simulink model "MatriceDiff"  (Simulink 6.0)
settings: Solver=ode45  StartTime=0  StopTime=17*t0  RelTol=1e-3
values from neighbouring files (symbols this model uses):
  b = S/Sm    (= 0.1)    [Constantes.m]    (also in ConstantesBck.m)
  beta = 0.95    [Constantes.m]    (also in ConstantesBck.m; ResCourV1.m = 1; ResCrV1.m = 1; ResEnerV1.m = 1)
  C = 1    [Constantes.m]    (also in ConstantesBck.m)
  gk = 36    [Constantes.m]    (also in ConstantesBck.m; sim_hh.m)
  gl = 0.3    [Constantes.m]    (also in ConstantesBck.m; sim_hh.m)
  gna = 120    [Constantes.m]    (also in ConstantesBck.m; sim_hh.m)
  h0 = 0.5961    [Constantes.m]    (also in ConstantesBck.m)
  m0 = 0.0529    [Constantes.m]    (also in ConstantesBck.m)
  mK = 0    [Constantes.m]    (also in ConstantesBck.m)
  mL = 0    [Constantes.m]    (also in ConstantesBck.m)
  mNa = 0    [Constantes.m]    (also in ConstantesBck.m)
  N = [6,8,5,5,7,1,2,6,9,1,1,9,4,8,8,7]    [Constantes.m]    (also in ConstantesBck.m; ImpedanceZtissus.m = 100; Ztissus.m = 100; charge.m = N(:,2))
  n0 = 0.3177    [Constantes.m]    (also in ConstantesBck.m)
  rapportIE = 10    [Constantes.m]
  Sm = 3.14e-2    (= 0.0314)    [Constantes.m]    (also in ConstantesBck.m = 0.000314)
  t0 = 2E-3    (= 0.002)    [Constantes.m]    (also in ConstantesBck.m = 0.001)
  Vk = -82    [Constantes.m]    (also in ConstantesBck.m)
  Vl = -59    [Constantes.m]    (also in ConstantesBck.m)
  Vna = 45    [Constantes.m]    (also in ConstantesBck.m)
  Vr = -70    [Constantes.m]    (also in ConstantesBck.m)
undefined symbols (not defined in the file or in its folder): ln
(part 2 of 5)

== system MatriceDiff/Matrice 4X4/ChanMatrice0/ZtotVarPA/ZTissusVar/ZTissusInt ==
  InStim : Inport  Orientation=down  Port=1  LatchInput=off
  VRefIn : Inport  Port=2  LatchInput=off
  Constant : Constant  Value=0
  Gain2 : Gain  Gain=-1
  Gain3 : Gain  Gain=-1
  Gain4 : Gain  Gain=-1
  Modele HH : Subsystem
  Modele HH1 : Subsystem
  Rint : Fcn  Expr=u*(1.6342*((abs(u)*1E6)^0.1267))*1E3/rapportIE
  Sum1 : Sum  Inputs=|+++
  Vout : Outport
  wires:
  Modele HH1/1(HHout) -> Gain3/1
  Modele HH/1(HHout) -> Gain4/1
  Rint/1 -> Sum1/2
  Gain2/1 -> Modele HH/1(HHin)
  InStim/1 -> Gain2/1, Rint/1, Modele HH1/1(HHin)
  Constant/1 -> Modele HH1/2(VRefIn)
  Sum1/1 -> Vout/1
  VRefIn/1 -> Modele HH/2(VRefIn)
  Gain3/1 -> Sum1/1
  Gain4/1 -> Sum1/3

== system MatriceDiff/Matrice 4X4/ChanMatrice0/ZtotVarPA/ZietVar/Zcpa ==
  InZcpa : Inport  Port=1  LatchInput=off
  Cdl : Fcn  Expr=u*1E9/(918.15-80.854*ln(abs(u)*1E6))
  Fcn : Fcn  Expr=u(1)^beta
  Transfer Fcn : TransferFcn  Denominator=[1 0]
  OutZcpa : Outport
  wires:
  Transfer Fcn/1 -> Fcn/1
  InZcpa/1 -> Cdl/1
  Fcn/1 -> OutZcpa/1
  Cdl/1 -> Transfer Fcn/1

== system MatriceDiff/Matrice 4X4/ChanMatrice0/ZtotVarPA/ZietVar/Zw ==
  InZw : Inport  Port=1  LatchInput=off
  Math Function : Math  Operator=sqrt
  Product : Product
  Transfer Fcn : TransferFcn  Numerator=[2]  Denominator=[1 0]
  sigma : Fcn  Expr=(67202-0.0688*((1E6*abs(u))^2)-11.273*(1E6*abs(u)))
  OutZw : Outport
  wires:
  Transfer Fcn/1 -> Math Function/1
  InZw/1 -> Transfer Fcn/1, sigma/1
  Math Function/1 -> Product/1
  sigma/1 -> Product/2
  Product/1 -> OutZw/1

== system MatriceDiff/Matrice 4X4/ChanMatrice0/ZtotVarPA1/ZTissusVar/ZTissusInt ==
  InStim : Inport  Orientation=down  Port=1  LatchInput=off
  VRefIn : Inport  Port=2  LatchInput=off
  Constant : Constant  Value=0
  Gain2 : Gain  Gain=-1
  Gain3 : Gain  Gain=-1
  Gain4 : Gain  Gain=-1
  Modele HH : Subsystem
  Modele HH1 : Subsystem
  Rint : Fcn  Expr=u*(1.6342*((abs(u)*1E6)^0.1267))*1E3/rapportIE
  Sum1 : Sum  Inputs=|+++
  Vout : Outport
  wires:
  Modele HH1/1(HHout) -> Gain3/1
  Modele HH/1(HHout) -> Gain4/1
  Rint/1 -> Sum1/2
  Gain2/1 -> Modele HH/1(HHin)
  InStim/1 -> Gain2/1, Rint/1, Modele HH1/1(HHin)
  Constant/1 -> Modele HH1/2(VRefIn)
  Sum1/1 -> Vout/1
  VRefIn/1 -> Modele HH/2(VRefIn)
  Gain3/1 -> Sum1/1
  Gain4/1 -> Sum1/3

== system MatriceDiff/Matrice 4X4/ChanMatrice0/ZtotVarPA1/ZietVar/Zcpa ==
  InZcpa : Inport  Port=1  LatchInput=off
  Cdl : Fcn  Expr=u*1E9/(918.15-80.854*ln(abs(u)*1E6))
  Fcn : Fcn  Expr=u(1)^beta
  Transfer Fcn : TransferFcn  Denominator=[1 0]
  OutZcpa : Outport
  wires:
  Transfer Fcn/1 -> Fcn/1
  InZcpa/1 -> Cdl/1
  Fcn/1 -> OutZcpa/1
  Cdl/1 -> Transfer Fcn/1

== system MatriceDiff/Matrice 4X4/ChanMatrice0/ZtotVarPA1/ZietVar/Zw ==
  InZw : Inport  Port=1  LatchInput=off
  Math Function : Math  Operator=sqrt
  Product : Product
  Transfer Fcn : TransferFcn  Numerator=[2]  Denominator=[1 0]
  sigma : Fcn  Expr=(67202-0.0688*((1E6*abs(u))^2)-11.273*(1E6*abs(u)))
  OutZw : Outport
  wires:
  Transfer Fcn/1 -> Math Function/1
  InZw/1 -> Transfer Fcn/1, sigma/1
  Math Function/1 -> Product/1
  sigma/1 -> Product/2
  Product/1 -> OutZw/1

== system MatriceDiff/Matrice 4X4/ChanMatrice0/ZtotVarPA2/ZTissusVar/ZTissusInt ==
  InStim : Inport  Orientation=down  Port=1  LatchInput=off
  VRefIn : Inport  Port=2  LatchInput=off
  Constant : Constant  Value=0
  Gain2 : Gain  Gain=-1
  Gain3 : Gain  Gain=-1
  Gain4 : Gain  Gain=-1
  Modele HH : Subsystem
  Modele HH1 : Subsystem
  Rint : Fcn  Expr=u*(1.6342*((abs(u)*1E6)^0.1267))*1E3/rapportIE
  Sum1 : Sum  Inputs=|+++
  Vout : Outport
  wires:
  Modele HH1/1(HHout) -> Gain3/1
  Modele HH/1(HHout) -> Gain4/1
  Rint/1 -> Sum1/2
  Gain2/1 -> Modele HH/1(HHin)
  InStim/1 -> Gain2/1, Rint/1, Modele HH1/1(HHin)
  Constant/1 -> Modele HH1/2(VRefIn)
  Sum1/1 -> Vout/1
  VRefIn/1 -> Modele HH/2(VRefIn)
  Gain3/1 -> Sum1/1
  Gain4/1 -> Sum1/3

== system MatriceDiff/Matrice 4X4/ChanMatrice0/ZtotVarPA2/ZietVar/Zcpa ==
  InZcpa : Inport  Port=1  LatchInput=off
  Cdl : Fcn  Expr=u*1E9/(918.15-80.854*ln(abs(u)*1E6))
  Fcn : Fcn  Expr=u(1)^beta
  Transfer Fcn : TransferFcn  Denominator=[1 0]
  OutZcpa : Outport
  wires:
  Transfer Fcn/1 -> Fcn/1
  InZcpa/1 -> Cdl/1
  Fcn/1 -> OutZcpa/1
  Cdl/1 -> Transfer Fcn/1

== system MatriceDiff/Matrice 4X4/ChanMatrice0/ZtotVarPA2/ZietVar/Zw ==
  InZw : Inport  Port=1  LatchInput=off
  Math Function : Math  Operator=sqrt
  Product : Product
  Transfer Fcn : TransferFcn  Numerator=[2]  Denominator=[1 0]
  sigma : Fcn  Expr=(67202-0.0688*((1E6*abs(u))^2)-11.273*(1E6*abs(u)))
  OutZw : Outport
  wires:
  Transfer Fcn/1 -> Math Function/1
  InZw/1 -> Transfer Fcn/1, sigma/1
  Math Function/1 -> Product/1
  sigma/1 -> Product/2
  Product/1 -> OutZw/1

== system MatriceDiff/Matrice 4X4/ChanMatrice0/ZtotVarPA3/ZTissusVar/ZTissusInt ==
  InStim : Inport  Orientation=down  Port=1  LatchInput=off
  VRefIn : Inport  Port=2  LatchInput=off
  Constant : Constant  Value=0
  Gain2 : Gain  Gain=-1
  Gain3 : Gain  Gain=-1
  Gain4 : Gain  Gain=-1
  Modele HH : Subsystem
  Modele HH1 : Subsystem
  Rint : Fcn  Expr=u*(1.6342*((abs(u)*1E6)^0.1267))*1E3/rapportIE
  Sum1 : Sum  Inputs=|+++
  Vout : Outport
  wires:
  Modele HH1/1(HHout) -> Gain3/1
  Modele HH/1(HHout) -> Gain4/1
  Rint/1 -> Sum1/2
  Gain2/1 -> Modele HH/1(HHin)
  InStim/1 -> Gain2/1, Rint/1, Modele HH1/1(HHin)
  Constant/1 -> Modele HH1/2(VRefIn)
  Sum1/1 -> Vout/1
  VRefIn/1 -> Modele HH/2(VRefIn)
  Gain3/1 -> Sum1/1
  Gain4/1 -> Sum1/3

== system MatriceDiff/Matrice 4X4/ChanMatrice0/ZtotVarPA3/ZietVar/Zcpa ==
  InZcpa : Inport  Port=1  LatchInput=off
  Cdl : Fcn  Expr=u*1E9/(918.15-80.854*ln(abs(u)*1E6))
  Fcn : Fcn  Expr=u(1)^beta
  Transfer Fcn : TransferFcn  Denominator=[1 0]
  OutZcpa : Outport
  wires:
  Transfer Fcn/1 -> Fcn/1
  InZcpa/1 -> Cdl/1
  Fcn/1 -> OutZcpa/1
  Cdl/1 -> Transfer Fcn/1

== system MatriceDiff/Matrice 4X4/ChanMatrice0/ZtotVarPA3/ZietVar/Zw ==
  InZw : Inport  Port=1  LatchInput=off
  Math Function : Math  Operator=sqrt
  Product : Product
  Transfer Fcn : TransferFcn  Numerator=[2]  Denominator=[1 0]
  sigma : Fcn  Expr=(67202-0.0688*((1E6*abs(u))^2)-11.273*(1E6*abs(u)))
  OutZw : Outport
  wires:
  Transfer Fcn/1 -> Math Function/1
  InZw/1 -> Transfer Fcn/1, sigma/1
  Math Function/1 -> Product/1
  sigma/1 -> Product/2
  Product/1 -> OutZw/1

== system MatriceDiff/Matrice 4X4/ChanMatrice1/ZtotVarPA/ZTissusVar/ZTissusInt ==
  InStim : Inport  Orientation=down  Port=1  LatchInput=off
  VRefIn : Inport  Port=2  LatchInput=off
  Constant : Constant  Value=0
  Gain2 : Gain  Gain=-1
  Gain3 : Gain  Gain=-1
  Gain4 : Gain  Gain=-1
  Modele HH : Subsystem
  Modele HH1 : Subsystem
  Rint : Fcn  Expr=u*(1.6342*((abs(u)*1E6)^0.1267))*1E3/rapportIE
  Sum1 : Sum  Inputs=|+++
  Vout : Outport
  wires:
  Modele HH1/1(HHout) -> Gain3/1
  Modele HH/1(HHout) -> Gain4/1
  Rint/1 -> Sum1/2
  Gain2/1 -> Modele HH/1(HHin)
  InStim/1 -> Gain2/1, Rint/1, Modele HH1/1(HHin)
  Constant/1 -> Modele HH1/2(VRefIn)
  Sum1/1 -> Vout/1
  VRefIn/1 -> Modele HH/2(VRefIn)
  Gain3/1 -> Sum1/1
  Gain4/1 -> Sum1/3

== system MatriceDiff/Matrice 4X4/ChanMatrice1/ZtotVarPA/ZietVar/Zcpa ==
  InZcpa : Inport  Port=1  LatchInput=off
  Cdl : Fcn  Expr=u*1E9/(918.15-80.854*ln(abs(u)*1E6))
  Fcn : Fcn  Expr=u(1)^beta
  Transfer Fcn : TransferFcn  Denominator=[1 0]
  OutZcpa : Outport
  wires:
  Transfer Fcn/1 -> Fcn/1
  InZcpa/1 -> Cdl/1
  Fcn/1 -> OutZcpa/1
  Cdl/1 -> Transfer Fcn/1

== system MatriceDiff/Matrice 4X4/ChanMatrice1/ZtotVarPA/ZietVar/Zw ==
  InZw : Inport  Port=1  LatchInput=off
  Math Function : Math  Operator=sqrt
  Product : Product
  Transfer Fcn : TransferFcn  Numerator=[2]  Denominator=[1 0]
  sigma : Fcn  Expr=(67202-0.0688*((1E6*abs(u))^2)-11.273*(1E6*abs(u)))
  OutZw : Outport
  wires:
  Transfer Fcn/1 -> Math Function/1
  InZw/1 -> Transfer Fcn/1, sigma/1
  Math Function/1 -> Product/1
  sigma/1 -> Product/2
  Product/1 -> OutZw/1

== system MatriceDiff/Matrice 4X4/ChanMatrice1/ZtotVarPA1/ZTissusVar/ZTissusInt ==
  InStim : Inport  Orientation=down  Port=1  LatchInput=off
  VRefIn : Inport  Port=2  LatchInput=off
  Constant : Constant  Value=0
  Gain2 : Gain  Gain=-1
  Gain3 : Gain  Gain=-1
  Gain4 : Gain  Gain=-1
  Modele HH : Subsystem
  Modele HH1 : Subsystem
  Rint : Fcn  Expr=u*(1.6342*((abs(u)*1E6)^0.1267))*1E3/rapportIE
  Sum1 : Sum  Inputs=|+++
  Vout : Outport
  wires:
  Modele HH1/1(HHout) -> Gain3/1
  Modele HH/1(HHout) -> Gain4/1
  Rint/1 -> Sum1/2
  Gain2/1 -> Modele HH/1(HHin)
  InStim/1 -> Gain2/1, Rint/1, Modele HH1/1(HHin)
  Constant/1 -> Modele HH1/2(VRefIn)
  Sum1/1 -> Vout/1
  VRefIn/1 -> Modele HH/2(VRefIn)
  Gain3/1 -> Sum1/1
  Gain4/1 -> Sum1/3

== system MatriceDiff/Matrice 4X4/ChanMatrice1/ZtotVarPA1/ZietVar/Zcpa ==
  InZcpa : Inport  Port=1  LatchInput=off
  Cdl : Fcn  Expr=u*1E9/(918.15-80.854*ln(abs(u)*1E6))
  Fcn : Fcn  Expr=u(1)^beta
  Transfer Fcn : TransferFcn  Denominator=[1 0]
  OutZcpa : Outport
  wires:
  Transfer Fcn/1 -> Fcn/1
  InZcpa/1 -> Cdl/1
  Fcn/1 -> OutZcpa/1
  Cdl/1 -> Transfer Fcn/1

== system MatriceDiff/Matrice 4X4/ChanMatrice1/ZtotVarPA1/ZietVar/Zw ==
  InZw : Inport  Port=1  LatchInput=off
  Math Function : Math  Operator=sqrt
  Product : Product
  Transfer Fcn : TransferFcn  Numerator=[2]  Denominator=[1 0]
  sigma : Fcn  Expr=(67202-0.0688*((1E6*abs(u))^2)-11.273*(1E6*abs(u)))
  OutZw : Outport
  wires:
  Transfer Fcn/1 -> Math Function/1
  InZw/1 -> Transfer Fcn/1, sigma/1
  Math Function/1 -> Product/1
  sigma/1 -> Product/2
  Product/1 -> OutZw/1

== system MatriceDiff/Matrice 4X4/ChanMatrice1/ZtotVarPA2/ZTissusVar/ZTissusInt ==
  InStim : Inport  Orientation=down  Port=1  LatchInput=off
  VRefIn : Inport  Port=2  LatchInput=off
  Constant : Constant  Value=0
  Gain2 : Gain  Gain=-1
  Gain3 : Gain  Gain=-1
  Gain4 : Gain  Gain=-1
  Modele HH : Subsystem
  Modele HH1 : Subsystem
  Rint : Fcn  Expr=u*(1.6342*((abs(u)*1E6)^0.1267))*1E3/rapportIE
  Sum1 : Sum  Inputs=|+++
  Vout : Outport
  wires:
  Modele HH1/1(HHout) -> Gain3/1
  Modele HH/1(HHout) -> Gain4/1
  Rint/1 -> Sum1/2
  Gain2/1 -> Modele HH/1(HHin)
  InStim/1 -> Gain2/1, Rint/1, Modele HH1/1(HHin)
  Constant/1 -> Modele HH1/2(VRefIn)
  Sum1/1 -> Vout/1
  VRefIn/1 -> Modele HH/2(VRefIn)
  Gain3/1 -> Sum1/1
  Gain4/1 -> Sum1/3

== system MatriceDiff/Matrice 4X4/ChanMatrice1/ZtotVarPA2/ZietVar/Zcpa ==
  InZcpa : Inport  Port=1  LatchInput=off
  Cdl : Fcn  Expr=u*1E9/(918.15-80.854*ln(abs(u)*1E6))
  Fcn : Fcn  Expr=u(1)^beta
  Transfer Fcn : TransferFcn  Denominator=[1 0]
  OutZcpa : Outport
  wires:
  Transfer Fcn/1 -> Fcn/1
  InZcpa/1 -> Cdl/1
  Fcn/1 -> OutZcpa/1
  Cdl/1 -> Transfer Fcn/1

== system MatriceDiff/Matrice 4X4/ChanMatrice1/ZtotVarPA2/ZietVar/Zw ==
  InZw : Inport  Port=1  LatchInput=off
  Math Function : Math  Operator=sqrt
  Product : Product
  Transfer Fcn : TransferFcn  Numerator=[2]  Denominator=[1 0]
  sigma : Fcn  Expr=(67202-0.0688*((1E6*abs(u))^2)-11.273*(1E6*abs(u)))
  OutZw : Outport
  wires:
  Transfer Fcn/1 -> Math Function/1
  InZw/1 -> Transfer Fcn/1, sigma/1
  Math Function/1 -> Product/1
  sigma/1 -> Product/2
  Product/1 -> OutZw/1

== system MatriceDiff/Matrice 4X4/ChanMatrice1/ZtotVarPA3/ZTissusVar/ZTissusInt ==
  InStim : Inport  Orientation=down  Port=1  LatchInput=off
  VRefIn : Inport  Port=2  LatchInput=off
  Constant : Constant  Value=0
  Gain2 : Gain  Gain=-1
  Gain3 : Gain  Gain=-1
  Gain4 : Gain  Gain=-1
  Modele HH : Subsystem
  Modele HH1 : Subsystem
  Rint : Fcn  Expr=u*(1.6342*((abs(u)*1E6)^0.1267))*1E3/rapportIE
  Sum1 : Sum  Inputs=|+++
  Vout : Outport
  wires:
  Modele HH1/1(HHout) -> Gain3/1
  Modele HH/1(HHout) -> Gain4/1
  Rint/1 -> Sum1/2
  Gain2/1 -> Modele HH/1(HHin)
  InStim/1 -> Gain2/1, Rint/1, Modele HH1/1(HHin)
  Constant/1 -> Modele HH1/2(VRefIn)
  Sum1/1 -> Vout/1
  VRefIn/1 -> Modele HH/2(VRefIn)
  Gain3/1 -> Sum1/1
  Gain4/1 -> Sum1/3

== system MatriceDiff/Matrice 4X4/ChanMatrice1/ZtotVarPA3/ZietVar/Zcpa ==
  InZcpa : Inport  Port=1  LatchInput=off
  Cdl : Fcn  Expr=u*1E9/(918.15-80.854*ln(abs(u)*1E6))
  Fcn : Fcn  Expr=u(1)^beta
  Transfer Fcn : TransferFcn  Denominator=[1 0]
  OutZcpa : Outport
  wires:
  Transfer Fcn/1 -> Fcn/1
  InZcpa/1 -> Cdl/1
  Fcn/1 -> OutZcpa/1
  Cdl/1 -> Transfer Fcn/1

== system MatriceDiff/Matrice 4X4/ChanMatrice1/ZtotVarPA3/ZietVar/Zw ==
  InZw : Inport  Port=1  LatchInput=off
  Math Function : Math  Operator=sqrt
  Product : Product
  Transfer Fcn : TransferFcn  Numerator=[2]  Denominator=[1 0]
  sigma : Fcn  Expr=(67202-0.0688*((1E6*abs(u))^2)-11.273*(1E6*abs(u)))
  OutZw : Outport
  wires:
  Transfer Fcn/1 -> Math Function/1
  InZw/1 -> Transfer Fcn/1, sigma/1
  Math Function/1 -> Product/1
  sigma/1 -> Product/2
  Product/1 -> OutZw/1

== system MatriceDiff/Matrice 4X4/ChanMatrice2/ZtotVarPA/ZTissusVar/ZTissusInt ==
  InStim : Inport  Orientation=down  Port=1  LatchInput=off
  VRefIn : Inport  Port=2  LatchInput=off
  Constant : Constant  Value=0
  Gain2 : Gain  Gain=-1
  Gain3 : Gain  Gain=-1
  Gain4 : Gain  Gain=-1
  Modele HH : Subsystem
  Modele HH1 : Subsystem
  Rint : Fcn  Expr=u*(1.6342*((abs(u)*1E6)^0.1267))*1E3/rapportIE
  Sum1 : Sum  Inputs=|+++
  Vout : Outport
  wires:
  Modele HH1/1(HHout) -> Gain3/1
  Modele HH/1(HHout) -> Gain4/1
  Rint/1 -> Sum1/2
  Gain2/1 -> Modele HH/1(HHin)
  InStim/1 -> Gain2/1, Rint/1, Modele HH1/1(HHin)
  Constant/1 -> Modele HH1/2(VRefIn)
  Sum1/1 -> Vout/1
  VRefIn/1 -> Modele HH/2(VRefIn)
  Gain3/1 -> Sum1/1
  Gain4/1 -> Sum1/3

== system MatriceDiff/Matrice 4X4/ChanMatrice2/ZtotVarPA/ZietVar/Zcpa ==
  InZcpa : Inport  Port=1  LatchInput=off
  Cdl : Fcn  Expr=u*1E9/(918.15-80.854*ln(abs(u)*1E6))
  Fcn : Fcn  Expr=u(1)^beta
  Transfer Fcn : TransferFcn  Denominator=[1 0]
  OutZcpa : Outport
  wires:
  Transfer Fcn/1 -> Fcn/1
  InZcpa/1 -> Cdl/1
  Fcn/1 -> OutZcpa/1
  Cdl/1 -> Transfer Fcn/1

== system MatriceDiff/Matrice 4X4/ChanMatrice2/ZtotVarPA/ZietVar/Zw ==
  InZw : Inport  Port=1  LatchInput=off
  Math Function : Math  Operator=sqrt
  Product : Product
  Transfer Fcn : TransferFcn  Numerator=[2]  Denominator=[1 0]
  sigma : Fcn  Expr=(67202-0.0688*((1E6*abs(u))^2)-11.273*(1E6*abs(u)))
  OutZw : Outport
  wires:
  Transfer Fcn/1 -> Math Function/1
  InZw/1 -> Transfer Fcn/1, sigma/1
  Math Function/1 -> Product/1
  sigma/1 -> Product/2
  Product/1 -> OutZw/1

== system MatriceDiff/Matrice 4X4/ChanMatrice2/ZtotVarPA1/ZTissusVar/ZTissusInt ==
  InStim : Inport  Orientation=down  Port=1  LatchInput=off
  VRefIn : Inport  Port=2  LatchInput=off
  Constant : Constant  Value=0
  Gain2 : Gain  Gain=-1
  Gain3 : Gain  Gain=-1
  Gain4 : Gain  Gain=-1
  Modele HH : Subsystem
  Modele HH1 : Subsystem
  Rint : Fcn  Expr=u*(1.6342*((abs(u)*1E6)^0.1267))*1E3/rapportIE
  Sum1 : Sum  Inputs=|+++
  Vout : Outport
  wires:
  Modele HH1/1(HHout) -> Gain3/1
  Modele HH/1(HHout) -> Gain4/1
  Rint/1 -> Sum1/2
  Gain2/1 -> Modele HH/1(HHin)
  InStim/1 -> Gain2/1, Rint/1, Modele HH1/1(HHin)
  Constant/1 -> Modele HH1/2(VRefIn)
  Sum1/1 -> Vout/1
  VRefIn/1 -> Modele HH/2(VRefIn)
  Gain3/1 -> Sum1/1
  Gain4/1 -> Sum1/3

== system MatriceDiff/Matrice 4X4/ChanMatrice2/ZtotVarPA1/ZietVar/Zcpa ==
  InZcpa : Inport  Port=1  LatchInput=off
  Cdl : Fcn  Expr=u*1E9/(918.15-80.854*ln(abs(u)*1E6))
  Fcn : Fcn  Expr=u(1)^beta
  Transfer Fcn : TransferFcn  Denominator=[1 0]
  OutZcpa : Outport
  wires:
  Transfer Fcn/1 -> Fcn/1
  InZcpa/1 -> Cdl/1
  Fcn/1 -> OutZcpa/1
  Cdl/1 -> Transfer Fcn/1

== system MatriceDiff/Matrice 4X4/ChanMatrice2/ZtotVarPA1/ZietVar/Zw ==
  InZw : Inport  Port=1  LatchInput=off
  Math Function : Math  Operator=sqrt
  Product : Product
  Transfer Fcn : TransferFcn  Numerator=[2]  Denominator=[1 0]
  sigma : Fcn  Expr=(67202-0.0688*((1E6*abs(u))^2)-11.273*(1E6*abs(u)))
  OutZw : Outport
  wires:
  Transfer Fcn/1 -> Math Function/1
  InZw/1 -> Transfer Fcn/1, sigma/1
  Math Function/1 -> Product/1
  sigma/1 -> Product/2
  Product/1 -> OutZw/1

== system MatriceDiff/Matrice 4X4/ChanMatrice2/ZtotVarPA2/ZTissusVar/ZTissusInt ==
  InStim : Inport  Orientation=down  Port=1  LatchInput=off
  VRefIn : Inport  Port=2  LatchInput=off
  Constant : Constant  Value=0
  Gain2 : Gain  Gain=-1
  Gain3 : Gain  Gain=-1
  Gain4 : Gain  Gain=-1
  Modele HH : Subsystem
  Modele HH1 : Subsystem
  Rint : Fcn  Expr=u*(1.6342*((abs(u)*1E6)^0.1267))*1E3/rapportIE
  Sum1 : Sum  Inputs=|+++
  Vout : Outport
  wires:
  Modele HH1/1(HHout) -> Gain3/1
  Modele HH/1(HHout) -> Gain4/1
  Rint/1 -> Sum1/2
  Gain2/1 -> Modele HH/1(HHin)
  InStim/1 -> Gain2/1, Rint/1, Modele HH1/1(HHin)
  Constant/1 -> Modele HH1/2(VRefIn)
  Sum1/1 -> Vout/1
  VRefIn/1 -> Modele HH/2(VRefIn)
  Gain3/1 -> Sum1/1
  Gain4/1 -> Sum1/3

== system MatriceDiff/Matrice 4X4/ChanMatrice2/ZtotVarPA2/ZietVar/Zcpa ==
  InZcpa : Inport  Port=1  LatchInput=off
  Cdl : Fcn  Expr=u*1E9/(918.15-80.854*ln(abs(u)*1E6))
  Fcn : Fcn  Expr=u(1)^beta
  Transfer Fcn : TransferFcn  Denominator=[1 0]
  OutZcpa : Outport
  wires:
  Transfer Fcn/1 -> Fcn/1
  InZcpa/1 -> Cdl/1
  Fcn/1 -> OutZcpa/1
  Cdl/1 -> Transfer Fcn/1

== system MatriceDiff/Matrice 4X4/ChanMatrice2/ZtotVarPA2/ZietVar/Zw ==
  InZw : Inport  Port=1  LatchInput=off
  Math Function : Math  Operator=sqrt
  Product : Product
  Transfer Fcn : TransferFcn  Numerator=[2]  Denominator=[1 0]
  sigma : Fcn  Expr=(67202-0.0688*((1E6*abs(u))^2)-11.273*(1E6*abs(u)))
  OutZw : Outport
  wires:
  Transfer Fcn/1 -> Math Function/1
  InZw/1 -> Transfer Fcn/1, sigma/1
  Math Function/1 -> Product/1
  sigma/1 -> Product/2
  Product/1 -> OutZw/1

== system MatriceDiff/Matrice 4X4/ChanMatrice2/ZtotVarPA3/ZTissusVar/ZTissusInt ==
  InStim : Inport  Orientation=down  Port=1  LatchInput=off
  VRefIn : Inport  Port=2  LatchInput=off
  Constant : Constant  Value=0
  Gain2 : Gain  Gain=-1
  Gain3 : Gain  Gain=-1
  Gain4 : Gain  Gain=-1
  Modele HH : Subsystem
  Modele HH1 : Subsystem
  Rint : Fcn  Expr=u*(1.6342*((abs(u)*1E6)^0.1267))*1E3/rapportIE
  Sum1 : Sum  Inputs=|+++
  Vout : Outport
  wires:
  Modele HH1/1(HHout) -> Gain3/1
  Modele HH/1(HHout) -> Gain4/1
  Rint/1 -> Sum1/2
  Gain2/1 -> Modele HH/1(HHin)
  InStim/1 -> Gain2/1, Rint/1, Modele HH1/1(HHin)
  Constant/1 -> Modele HH1/2(VRefIn)
  Sum1/1 -> Vout/1
  VRefIn/1 -> Modele HH/2(VRefIn)
  Gain3/1 -> Sum1/1
  Gain4/1 -> Sum1/3

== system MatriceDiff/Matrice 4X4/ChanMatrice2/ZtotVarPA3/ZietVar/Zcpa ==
  InZcpa : Inport  Port=1  LatchInput=off
  Cdl : Fcn  Expr=u*1E9/(918.15-80.854*ln(abs(u)*1E6))
  Fcn : Fcn  Expr=u(1)^beta
  Transfer Fcn : TransferFcn  Denominator=[1 0]
  OutZcpa : Outport
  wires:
  Transfer Fcn/1 -> Fcn/1
  InZcpa/1 -> Cdl/1
  Fcn/1 -> OutZcpa/1
  Cdl/1 -> Transfer Fcn/1

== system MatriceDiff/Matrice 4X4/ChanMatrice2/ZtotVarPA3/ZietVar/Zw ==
  InZw : Inport  Port=1  LatchInput=off
  Math Function : Math  Operator=sqrt
  Product : Product
  Transfer Fcn : TransferFcn  Numerator=[2]  Denominator=[1 0]
  sigma : Fcn  Expr=(67202-0.0688*((1E6*abs(u))^2)-11.273*(1E6*abs(u)))
  OutZw : Outport
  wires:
  Transfer Fcn/1 -> Math Function/1
  InZw/1 -> Transfer Fcn/1, sigma/1
  Math Function/1 -> Product/1
  sigma/1 -> Product/2
  Product/1 -> OutZw/1

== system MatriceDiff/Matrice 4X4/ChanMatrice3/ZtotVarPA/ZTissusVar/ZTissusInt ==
  InStim : Inport  Orientation=down  Port=1  LatchInput=off
  VRefIn : Inport  Port=2  LatchInput=off
  Constant : Constant  Value=0
  Gain2 : Gain  Gain=-1
  Gain3 : Gain  Gain=-1
  Gain4 : Gain  Gain=-1
  Modele HH : Subsystem
  Modele HH1 : Subsystem
  Rint : Fcn  Expr=u*(1.6342*((abs(u)*1E6)^0.1267))*1E3/rapportIE
  Sum1 : Sum  Inputs=|+++
  Vout : Outport
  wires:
  Modele HH1/1(HHout) -> Gain3/1
  Modele HH/1(HHout) -> Gain4/1
  Rint/1 -> Sum1/2
  Gain2/1 -> Modele HH/1(HHin)
  InStim/1 -> Gain2/1, Rint/1, Modele HH1/1(HHin)
  Constant/1 -> Modele HH1/2(VRefIn)
  Sum1/1 -> Vout/1
  VRefIn/1 -> Modele HH/2(VRefIn)
  Gain3/1 -> Sum1/1
  Gain4/1 -> Sum1/3

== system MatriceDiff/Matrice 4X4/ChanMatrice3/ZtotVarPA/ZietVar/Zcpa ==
  InZcpa : Inport  Port=1  LatchInput=off
  Cdl : Fcn  Expr=u*1E9/(918.15-80.854*ln(abs(u)*1E6))
  Fcn : Fcn  Expr=u(1)^beta
  Transfer Fcn : TransferFcn  Denominator=[1 0]
  OutZcpa : Outport
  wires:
  Transfer Fcn/1 -> Fcn/1
  InZcpa/1 -> Cdl/1
  Fcn/1 -> OutZcpa/1
  Cdl/1 -> Transfer Fcn/1

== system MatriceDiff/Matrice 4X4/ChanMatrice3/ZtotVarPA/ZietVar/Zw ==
  InZw : Inport  Port=1  LatchInput=off
  Math Function : Math  Operator=sqrt
  Product : Product
  Transfer Fcn : TransferFcn  Numerator=[2]  Denominator=[1 0]
  sigma : Fcn  Expr=(67202-0.0688*((1E6*abs(u))^2)-11.273*(1E6*abs(u)))
  OutZw : Outport
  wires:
  Transfer Fcn/1 -> Math Function/1
  InZw/1 -> Transfer Fcn/1, sigma/1
  Math Function/1 -> Product/1
  sigma/1 -> Product/2
  Product/1 -> OutZw/1

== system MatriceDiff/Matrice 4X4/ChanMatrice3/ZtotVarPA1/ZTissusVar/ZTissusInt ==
  InStim : Inport  Orientation=down  Port=1  LatchInput=off
  VRefIn : Inport  Port=2  LatchInput=off
  Constant : Constant  Value=0
  Gain2 : Gain  Gain=-1
  Gain3 : Gain  Gain=-1
  Gain4 : Gain  Gain=-1
  Modele HH : Subsystem
  Modele HH1 : Subsystem
  Rint : Fcn  Expr=u*(1.6342*((abs(u)*1E6)^0.1267))*1E3/rapportIE
  Sum1 : Sum  Inputs=|+++
  Vout : Outport
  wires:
  Modele HH1/1(HHout) -> Gain3/1
  Modele HH/1(HHout) -> Gain4/1
  Rint/1 -> Sum1/2
  Gain2/1 -> Modele HH/1(HHin)
  InStim/1 -> Gain2/1, Rint/1, Modele HH1/1(HHin)
  Constant/1 -> Modele HH1/2(VRefIn)
  Sum1/1 -> Vout/1
  VRefIn/1 -> Modele HH/2(VRefIn)
  Gain3/1 -> Sum1/1
  Gain4/1 -> Sum1/3

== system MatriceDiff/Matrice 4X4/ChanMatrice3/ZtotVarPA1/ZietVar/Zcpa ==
  InZcpa : Inport  Port=1  LatchInput=off
  Cdl : Fcn  Expr=u*1E9/(918.15-80.854*ln(abs(u)*1E6))
  Fcn : Fcn  Expr=u(1)^beta
  Transfer Fcn : TransferFcn  Denominator=[1 0]
  OutZcpa : Outport
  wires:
  Transfer Fcn/1 -> Fcn/1
  InZcpa/1 -> Cdl/1
  Fcn/1 -> OutZcpa/1
  Cdl/1 -> Transfer Fcn/1

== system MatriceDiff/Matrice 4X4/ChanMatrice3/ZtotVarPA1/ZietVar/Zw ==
  InZw : Inport  Port=1  LatchInput=off
  Math Function : Math  Operator=sqrt
  Product : Product
  Transfer Fcn : TransferFcn  Numerator=[2]  Denominator=[1 0]
  sigma : Fcn  Expr=(67202-0.0688*((1E6*abs(u))^2)-11.273*(1E6*abs(u)))
  OutZw : Outport
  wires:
  Transfer Fcn/1 -> Math Function/1
  InZw/1 -> Transfer Fcn/1, sigma/1
  Math Function/1 -> Product/1
  sigma/1 -> Product/2
  Product/1 -> OutZw/1

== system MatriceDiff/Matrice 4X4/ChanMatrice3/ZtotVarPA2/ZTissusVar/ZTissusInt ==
  InStim : Inport  Orientation=down  Port=1  LatchInput=off
  VRefIn : Inport  Port=2  LatchInput=off
  Constant : Constant  Value=0
  Gain2 : Gain  Gain=-1
  Gain3 : Gain  Gain=-1
  Gain4 : Gain  Gain=-1
  Modele HH : Subsystem
  Modele HH1 : Subsystem
  Rint : Fcn  Expr=u*(1.6342*((abs(u)*1E6)^0.1267))*1E3/rapportIE
  Sum1 : Sum  Inputs=|+++
  Vout : Outport
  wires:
  Modele HH1/1(HHout) -> Gain3/1
  Modele HH/1(HHout) -> Gain4/1
  Rint/1 -> Sum1/2
  Gain2/1 -> Modele HH/1(HHin)
  InStim/1 -> Gain2/1, Rint/1, Modele HH1/1(HHin)
  Constant/1 -> Modele HH1/2(VRefIn)
  Sum1/1 -> Vout/1
  VRefIn/1 -> Modele HH/2(VRefIn)
  Gain3/1 -> Sum1/1
  Gain4/1 -> Sum1/3

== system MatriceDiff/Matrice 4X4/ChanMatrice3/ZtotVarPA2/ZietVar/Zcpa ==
  InZcpa : Inport  Port=1  LatchInput=off
  Cdl : Fcn  Expr=u*1E9/(918.15-80.854*ln(abs(u)*1E6))
  Fcn : Fcn  Expr=u(1)^beta
  Transfer Fcn : TransferFcn  Denominator=[1 0]
  OutZcpa : Outport
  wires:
  Transfer Fcn/1 -> Fcn/1
  InZcpa/1 -> Cdl/1
  Fcn/1 -> OutZcpa/1
  Cdl/1 -> Transfer Fcn/1

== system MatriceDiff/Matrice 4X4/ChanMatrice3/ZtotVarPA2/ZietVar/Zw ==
  InZw : Inport  Port=1  LatchInput=off
  Math Function : Math  Operator=sqrt
  Product : Product
  Transfer Fcn : TransferFcn  Numerator=[2]  Denominator=[1 0]
  sigma : Fcn  Expr=(67202-0.0688*((1E6*abs(u))^2)-11.273*(1E6*abs(u)))
  OutZw : Outport
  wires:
  Transfer Fcn/1 -> Math Function/1
  InZw/1 -> Transfer Fcn/1, sigma/1
  Math Function/1 -> Product/1
  sigma/1 -> Product/2
  Product/1 -> OutZw/1

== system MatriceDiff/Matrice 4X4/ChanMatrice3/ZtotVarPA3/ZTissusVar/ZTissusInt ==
  InStim : Inport  Orientation=down  Port=1  LatchInput=off
  VRefIn : Inport  Port=2  LatchInput=off
  Constant : Constant  Value=0
  Gain2 : Gain  Gain=-1
  Gain3 : Gain  Gain=-1
  Gain4 : Gain  Gain=-1
  Modele HH : Subsystem
  Modele HH1 : Subsystem
  Rint : Fcn  Expr=u*(1.6342*((abs(u)*1E6)^0.1267))*1E3/rapportIE
  Sum1 : Sum  Inputs=|+++
  Vout : Outport
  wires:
  Modele HH1/1(HHout) -> Gain3/1
  Modele HH/1(HHout) -> Gain4/1
  Rint/1 -> Sum1/2
  Gain2/1 -> Modele HH/1(HHin)
  InStim/1 -> Gain2/1, Rint/1, Modele HH1/1(HHin)
  Constant/1 -> Modele HH1/2(VRefIn)
  Sum1/1 -> Vout/1
  VRefIn/1 -> Modele HH/2(VRefIn)
  Gain3/1 -> Sum1/1
  Gain4/1 -> Sum1/3

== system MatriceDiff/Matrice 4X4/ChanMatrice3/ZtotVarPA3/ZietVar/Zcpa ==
  InZcpa : Inport  Port=1  LatchInput=off
  Cdl : Fcn  Expr=u*1E9/(918.15-80.854*ln(abs(u)*1E6))
  Fcn : Fcn  Expr=u(1)^beta
  Transfer Fcn : TransferFcn  Denominator=[1 0]
  OutZcpa : Outport
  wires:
  Transfer Fcn/1 -> Fcn/1
  InZcpa/1 -> Cdl/1
  Fcn/1 -> OutZcpa/1
  Cdl/1 -> Transfer Fcn/1

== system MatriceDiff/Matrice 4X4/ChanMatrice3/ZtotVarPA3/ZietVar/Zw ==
  InZw : Inport  Port=1  LatchInput=off
  Math Function : Math  Operator=sqrt
  Product : Product
  Transfer Fcn : TransferFcn  Numerator=[2]  Denominator=[1 0]
  sigma : Fcn  Expr=(67202-0.0688*((1E6*abs(u))^2)-11.273*(1E6*abs(u)))
  OutZw : Outport
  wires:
  Transfer Fcn/1 -> Math Function/1
  InZw/1 -> Transfer Fcn/1, sigma/1
  Math Function/1 -> Product/1
  sigma/1 -> Product/2
  Product/1 -> OutZw/1

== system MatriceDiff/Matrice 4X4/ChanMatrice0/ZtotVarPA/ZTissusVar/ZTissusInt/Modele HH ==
  HHin : Inport  Port=1  LatchInput=off
  VRefIn : Inport  Port=2  LatchInput=off
  FK : Subsystem
  FL : Fcn  Expr=gl*(u-Vl)
  FNa : Subsystem
  Gain : Gain  Gain=(1-b)/C
  Gain1 : Gain  Gain=1/(Sm*(1-b))
  Gain2 : Gain  Gain=1+mK*(b/(1-b))
  Gain3 : Gain  Gain=1+mL*(b/(1-b))
  Gain4 : Gain  Gain=1+mNa*(b/(1-b))
  Integrator : Integrator  InitialCondition=Vr
  Sum : Sum  Inputs=|---+
  Sum1 : Sum  Inputs=|+-
  HHout : Outport
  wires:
  Sum/1 -> Gain/1
  Gain/1 -> Integrator/1
  FK/1(FKout) -> Gain4/1
  FNa/1(FNaOut) -> Gain2/1
  FL/1 -> Gain3/1
  HHin/1 -> Gain1/1
  Integrator/1 -> Sum1/1
  Sum1/1 -> HHout/1, FNa/1(FNaIn), FL/1, FK/1(FKIn)
  VRefIn/1 -> Sum1/2
  Gain1/1 -> Sum/4
  Gain4/1 -> Sum/1
  Gain2/1 -> Sum/2
  Gain3/1 -> Sum/3

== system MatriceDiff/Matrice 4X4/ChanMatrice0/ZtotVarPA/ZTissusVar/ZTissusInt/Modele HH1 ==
  HHin : Inport  Port=1  LatchInput=off
  VRefIn : Inport  Port=2  LatchInput=off
  FK : Subsystem
  FL : Fcn  Expr=gl*(u-Vl)
  FNa : Subsystem
  Gain : Gain  Gain=(1-b)/C
  Gain1 : Gain  Gain=1/(Sm*(1-b))
  Gain2 : Gain  Gain=1+mK*(b/(1-b))
  Gain3 : Gain  Gain=1+mL*(b/(1-b))
  Gain4 : Gain  Gain=1+mNa*(b/(1-b))
  Integrator : Integrator  InitialCondition=Vr
  Sum : Sum  Inputs=|---+
  Sum1 : Sum  Inputs=|++
  HHout : Outport
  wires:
  Sum/1 -> Gain/1
  Gain/1 -> Integrator/1
  FK/1(FKout) -> Gain4/1
  FNa/1(FNaOut) -> Gain2/1
  FL/1 -> Gain3/1
  HHin/1 -> Gain1/1
  Integrator/1 -> Sum1/1
  Sum1/1 -> HHout/1, FNa/1(FNaIn), FL/1, FK/1(FKIn)
  VRefIn/1 -> Sum1/2
  Gain1/1 -> Sum/4
  Gain4/1 -> Sum/1
  Gain2/1 -> Sum/2
  Gain3/1 -> Sum/3

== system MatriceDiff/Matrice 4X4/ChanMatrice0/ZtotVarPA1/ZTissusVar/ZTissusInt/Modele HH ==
  HHin : Inport  Port=1  LatchInput=off
  VRefIn : Inport  Port=2  LatchInput=off
  FK : Subsystem
  FL : Fcn  Expr=gl*(u-Vl)
  FNa : Subsystem
  Gain : Gain  Gain=(1-b)/C
  Gain1 : Gain  Gain=1/(Sm*(1-b))
  Gain2 : Gain  Gain=1+mK*(b/(1-b))
  Gain3 : Gain  Gain=1+mL*(b/(1-b))
  Gain4 : Gain  Gain=1+mNa*(b/(1-b))
  Integrator : Integrator  InitialCondition=Vr
  Sum : Sum  Inputs=|---+
  Sum1 : Sum  Inputs=|+-
  HHout : Outport
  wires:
  Sum/1 -> Gain/1
  Gain/1 -> Integrator/1
  FK/1(FKout) -> Gain4/1
  FNa/1(FNaOut) -> Gain2/1
  FL/1 -> Gain3/1
  HHin/1 -> Gain1/1
  Integrator/1 -> Sum1/1
  Sum1/1 -> HHout/1, FNa/1(FNaIn), FL/1, FK/1(FKIn)
  VRefIn/1 -> Sum1/2
  Gain1/1 -> Sum/4
  Gain4/1 -> Sum/1
  Gain2/1 -> Sum/2
  Gain3/1 -> Sum/3

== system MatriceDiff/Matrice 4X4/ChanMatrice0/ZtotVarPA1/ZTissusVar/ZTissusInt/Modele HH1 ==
  HHin : Inport  Port=1  LatchInput=off
  VRefIn : Inport  Port=2  LatchInput=off
  FK : Subsystem
  FL : Fcn  Expr=gl*(u-Vl)
  FNa : Subsystem
  Gain : Gain  Gain=(1-b)/C
  Gain1 : Gain  Gain=1/(Sm*(1-b))
  Gain2 : Gain  Gain=1+mK*(b/(1-b))
  Gain3 : Gain  Gain=1+mL*(b/(1-b))
  Gain4 : Gain  Gain=1+mNa*(b/(1-b))
  Integrator : Integrator  InitialCondition=Vr
  Sum : Sum  Inputs=|---+
  Sum1 : Sum  Inputs=|++
  HHout : Outport
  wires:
  Sum/1 -> Gain/1
  Gain/1 -> Integrator/1
  FK/1(FKout) -> Gain4/1
  FNa/1(FNaOut) -> Gain2/1
  FL/1 -> Gain3/1
  HHin/1 -> Gain1/1
  Integrator/1 -> Sum1/1
  Sum1/1 -> HHout/1, FNa/1(FNaIn), FL/1, FK/1(FKIn)
  VRefIn/1 -> Sum1/2
  Gain1/1 -> Sum/4
  Gain4/1 -> Sum/1
  Gain2/1 -> Sum/2
  Gain3/1 -> Sum/3

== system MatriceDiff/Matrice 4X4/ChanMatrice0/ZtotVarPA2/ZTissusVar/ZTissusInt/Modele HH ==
  HHin : Inport  Port=1  LatchInput=off
  VRefIn : Inport  Port=2  LatchInput=off
  FK : Subsystem
  FL : Fcn  Expr=gl*(u-Vl)
  FNa : Subsystem
  Gain : Gain  Gain=(1-b)/C
  Gain1 : Gain  Gain=1/(Sm*(1-b))
  Gain2 : Gain  Gain=1+mK*(b/(1-b))
  Gain3 : Gain  Gain=1+mL*(b/(1-b))
  Gain4 : Gain  Gain=1+mNa*(b/(1-b))
  Integrator : Integrator  InitialCondition=Vr
  Sum : Sum  Inputs=|---+
  Sum1 : Sum  Inputs=|+-
  HHout : Outport
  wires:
  Sum/1 -> Gain/1
  Gain/1 -> Integrator/1
  FK/1(FKout) -> Gain4/1
  FNa/1(FNaOut) -> Gain2/1
  FL/1 -> Gain3/1
  HHin/1 -> Gain1/1
  Integrator/1 -> Sum1/1
  Sum1/1 -> HHout/1, FNa/1(FNaIn), FL/1, FK/1(FKIn)
  VRefIn/1 -> Sum1/2
  Gain1/1 -> Sum/4
  Gain4/1 -> Sum/1
  Gain2/1 -> Sum/2
  Gain3/1 -> Sum/3

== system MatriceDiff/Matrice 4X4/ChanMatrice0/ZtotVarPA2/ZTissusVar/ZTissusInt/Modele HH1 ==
  HHin : Inport  Port=1  LatchInput=off
  VRefIn : Inport  Port=2  LatchInput=off
  FK : Subsystem
  FL : Fcn  Expr=gl*(u-Vl)
  FNa : Subsystem
  Gain : Gain  Gain=(1-b)/C
  Gain1 : Gain  Gain=1/(Sm*(1-b))
  Gain2 : Gain  Gain=1+mK*(b/(1-b))
  Gain3 : Gain  Gain=1+mL*(b/(1-b))
  Gain4 : Gain  Gain=1+mNa*(b/(1-b))
  Integrator : Integrator  InitialCondition=Vr
  Sum : Sum  Inputs=|---+
  Sum1 : Sum  Inputs=|++
  HHout : Outport
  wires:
  Sum/1 -> Gain/1
  Gain/1 -> Integrator/1
  FK/1(FKout) -> Gain4/1
  FNa/1(FNaOut) -> Gain2/1
  FL/1 -> Gain3/1
  HHin/1 -> Gain1/1
  Integrator/1 -> Sum1/1
  Sum1/1 -> HHout/1, FNa/1(FNaIn), FL/1, FK/1(FKIn)
  VRefIn/1 -> Sum1/2
  Gain1/1 -> Sum/4
  Gain4/1 -> Sum/1
  Gain2/1 -> Sum/2
  Gain3/1 -> Sum/3

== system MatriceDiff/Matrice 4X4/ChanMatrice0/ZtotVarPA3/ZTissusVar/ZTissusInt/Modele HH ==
  HHin : Inport  Port=1  LatchInput=off
  VRefIn : Inport  Port=2  LatchInput=off
  FK : Subsystem
  FL : Fcn  Expr=gl*(u-Vl)
  FNa : Subsystem
  Gain : Gain  Gain=(1-b)/C
  Gain1 : Gain  Gain=1/(Sm*(1-b))
  Gain2 : Gain  Gain=1+mK*(b/(1-b))
  Gain3 : Gain  Gain=1+mL*(b/(1-b))
  Gain4 : Gain  Gain=1+mNa*(b/(1-b))
  Integrator : Integrator  InitialCondition=Vr
  Sum : Sum  Inputs=|---+
  Sum1 : Sum  Inputs=|+-
  HHout : Outport
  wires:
  Sum/1 -> Gain/1
  Gain/1 -> Integrator/1
  FK/1(FKout) -> Gain4/1
  FNa/1(FNaOut) -> Gain2/1
  FL/1 -> Gain3/1
  HHin/1 -> Gain1/1
  Integrator/1 -> Sum1/1
  Sum1/1 -> HHout/1, FNa/1(FNaIn), FL/1, FK/1(FKIn)
  VRefIn/1 -> Sum1/2
  Gain1/1 -> Sum/4
  Gain4/1 -> Sum/1
  Gain2/1 -> Sum/2
  Gain3/1 -> Sum/3

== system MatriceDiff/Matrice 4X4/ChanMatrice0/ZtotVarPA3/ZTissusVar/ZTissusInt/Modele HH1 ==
  HHin : Inport  Port=1  LatchInput=off
  VRefIn : Inport  Port=2  LatchInput=off
  FK : Subsystem
  FL : Fcn  Expr=gl*(u-Vl)
  FNa : Subsystem
  Gain : Gain  Gain=(1-b)/C
  Gain1 : Gain  Gain=1/(Sm*(1-b))
  Gain2 : Gain  Gain=1+mK*(b/(1-b))
  Gain3 : Gain  Gain=1+mL*(b/(1-b))
  Gain4 : Gain  Gain=1+mNa*(b/(1-b))
  Integrator : Integrator  InitialCondition=Vr
  Sum : Sum  Inputs=|---+
  Sum1 : Sum  Inputs=|++
  HHout : Outport
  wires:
  Sum/1 -> Gain/1
  Gain/1 -> Integrator/1
  FK/1(FKout) -> Gain4/1
  FNa/1(FNaOut) -> Gain2/1
  FL/1 -> Gain3/1
  HHin/1 -> Gain1/1
  Integrator/1 -> Sum1/1
  Sum1/1 -> HHout/1, FNa/1(FNaIn), FL/1, FK/1(FKIn)
  VRefIn/1 -> Sum1/2
  Gain1/1 -> Sum/4
  Gain4/1 -> Sum/1
  Gain2/1 -> Sum/2
  Gain3/1 -> Sum/3

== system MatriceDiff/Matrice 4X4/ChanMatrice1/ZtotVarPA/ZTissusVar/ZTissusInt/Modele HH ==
  HHin : Inport  Port=1  LatchInput=off
  VRefIn : Inport  Port=2  LatchInput=off
  FK : Subsystem
  FL : Fcn  Expr=gl*(u-Vl)
  FNa : Subsystem
  Gain : Gain  Gain=(1-b)/C
  Gain1 : Gain  Gain=1/(Sm*(1-b))
  Gain2 : Gain  Gain=1+mK*(b/(1-b))
  Gain3 : Gain  Gain=1+mL*(b/(1-b))
  Gain4 : Gain  Gain=1+mNa*(b/(1-b))
  Integrator : Integrator  InitialCondition=Vr
  Sum : Sum  Inputs=|---+
  Sum1 : Sum  Inputs=|+-
  HHout : Outport
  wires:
  Sum/1 -> Gain/1
  Gain/1 -> Integrator/1
  FK/1(FKout) -> Gain4/1
  FNa/1(FNaOut) -> Gain2/1
  FL/1 -> Gain3/1
  HHin/1 -> Gain1/1
  Integrator/1 -> Sum1/1
  Sum1/1 -> HHout/1, FNa/1(FNaIn), FL/1, FK/1(FKIn)
  VRefIn/1 -> Sum1/2
  Gain1/1 -> Sum/4
  Gain4/1 -> Sum/1
  Gain2/1 -> Sum/2
  Gain3/1 -> Sum/3

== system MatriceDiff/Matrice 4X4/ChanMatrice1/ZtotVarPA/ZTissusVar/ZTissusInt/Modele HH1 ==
  HHin : Inport  Port=1  LatchInput=off
  VRefIn : Inport  Port=2  LatchInput=off
  FK : Subsystem
  FL : Fcn  Expr=gl*(u-Vl)
  FNa : Subsystem
  Gain : Gain  Gain=(1-b)/C
  Gain1 : Gain  Gain=1/(Sm*(1-b))
  Gain2 : Gain  Gain=1+mK*(b/(1-b))
  Gain3 : Gain  Gain=1+mL*(b/(1-b))
  Gain4 : Gain  Gain=1+mNa*(b/(1-b))
  Integrator : Integrator  InitialCondition=Vr
  Sum : Sum  Inputs=|---+
  Sum1 : Sum  Inputs=|++
  HHout : Outport
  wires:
  Sum/1 -> Gain/1
  Gain/1 -> Integrator/1
  FK/1(FKout) -> Gain4/1
  FNa/1(FNaOut) -> Gain2/1
  FL/1 -> Gain3/1
  HHin/1 -> Gain1/1
  Integrator/1 -> Sum1/1
  Sum1/1 -> HHout/1, FNa/1(FNaIn), FL/1, FK/1(FKIn)
  VRefIn/1 -> Sum1/2
  Gain1/1 -> Sum/4
  Gain4/1 -> Sum/1
  Gain2/1 -> Sum/2
  Gain3/1 -> Sum/3

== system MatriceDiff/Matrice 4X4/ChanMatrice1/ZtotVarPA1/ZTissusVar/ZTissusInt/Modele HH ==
  HHin : Inport  Port=1  LatchInput=off
  VRefIn : Inport  Port=2  LatchInput=off
  FK : Subsystem
  FL : Fcn  Expr=gl*(u-Vl)
  FNa : Subsystem
  Gain : Gain  Gain=(1-b)/C
  Gain1 : Gain  Gain=1/(Sm*(1-b))
  Gain2 : Gain  Gain=1+mK*(b/(1-b))
  Gain3 : Gain  Gain=1+mL*(b/(1-b))
  Gain4 : Gain  Gain=1+mNa*(b/(1-b))
  Integrator : Integrator  InitialCondition=Vr
  Sum : Sum  Inputs=|---+
  Sum1 : Sum  Inputs=|+-
  HHout : Outport
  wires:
  Sum/1 -> Gain/1
  Gain/1 -> Integrator/1
  FK/1(FKout) -> Gain4/1
  FNa/1(FNaOut) -> Gain2/1
  FL/1 -> Gain3/1
  HHin/1 -> Gain1/1
  Integrator/1 -> Sum1/1
  Sum1/1 -> HHout/1, FNa/1(FNaIn), FL/1, FK/1(FKIn)
  VRefIn/1 -> Sum1/2
  Gain1/1 -> Sum/4
  Gain4/1 -> Sum/1
  Gain2/1 -> Sum/2
  Gain3/1 -> Sum/3

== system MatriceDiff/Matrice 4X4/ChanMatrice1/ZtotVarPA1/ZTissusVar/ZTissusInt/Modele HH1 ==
  HHin : Inport  Port=1  LatchInput=off
  VRefIn : Inport  Port=2  LatchInput=off
  FK : Subsystem
  FL : Fcn  Expr=gl*(u-Vl)
  FNa : Subsystem
  Gain : Gain  Gain=(1-b)/C
  Gain1 : Gain  Gain=1/(Sm*(1-b))
  Gain2 : Gain  Gain=1+mK*(b/(1-b))
  Gain3 : Gain  Gain=1+mL*(b/(1-b))
  Gain4 : Gain  Gain=1+mNa*(b/(1-b))
  Integrator : Integrator  InitialCondition=Vr
  Sum : Sum  Inputs=|---+
  Sum1 : Sum  Inputs=|++
  HHout : Outport
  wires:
  Sum/1 -> Gain/1
  Gain/1 -> Integrator/1
  FK/1(FKout) -> Gain4/1
  FNa/1(FNaOut) -> Gain2/1
  FL/1 -> Gain3/1
  HHin/1 -> Gain1/1
  Integrator/1 -> Sum1/1
  Sum1/1 -> HHout/1, FNa/1(FNaIn), FL/1, FK/1(FKIn)
  VRefIn/1 -> Sum1/2
  Gain1/1 -> Sum/4
  Gain4/1 -> Sum/1
  Gain2/1 -> Sum/2
  Gain3/1 -> Sum/3

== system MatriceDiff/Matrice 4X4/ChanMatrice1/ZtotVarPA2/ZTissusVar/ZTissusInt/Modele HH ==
  HHin : Inport  Port=1  LatchInput=off
  VRefIn : Inport  Port=2  LatchInput=off
  FK : Subsystem
  FL : Fcn  Expr=gl*(u-Vl)
  FNa : Subsystem
  Gain : Gain  Gain=(1-b)/C
  Gain1 : Gain  Gain=1/(Sm*(1-b))
  Gain2 : Gain  Gain=1+mK*(b/(1-b))
  Gain3 : Gain  Gain=1+mL*(b/(1-b))
  Gain4 : Gain  Gain=1+mNa*(b/(1-b))
  Integrator : Integrator  InitialCondition=Vr
  Sum : Sum  Inputs=|---+
  Sum1 : Sum  Inputs=|+-
  HHout : Outport
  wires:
  Sum/1 -> Gain/1
  Gain/1 -> Integrator/1
  FK/1(FKout) -> Gain4/1
  FNa/1(FNaOut) -> Gain2/1
  FL/1 -> Gain3/1
  HHin/1 -> Gain1/1
  Integrator/1 -> Sum1/1
  Sum1/1 -> HHout/1, FNa/1(FNaIn), FL/1, FK/1(FKIn)
  VRefIn/1 -> Sum1/2
  Gain1/1 -> Sum/4
  Gain4/1 -> Sum/1
  Gain2/1 -> Sum/2
  Gain3/1 -> Sum/3

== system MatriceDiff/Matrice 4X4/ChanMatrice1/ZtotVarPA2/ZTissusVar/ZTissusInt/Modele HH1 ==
  HHin : Inport  Port=1  LatchInput=off
  VRefIn : Inport  Port=2  LatchInput=off
  FK : Subsystem
  FL : Fcn  Expr=gl*(u-Vl)
  FNa : Subsystem
  Gain : Gain  Gain=(1-b)/C
  Gain1 : Gain  Gain=1/(Sm*(1-b))
  Gain2 : Gain  Gain=1+mK*(b/(1-b))
  Gain3 : Gain  Gain=1+mL*(b/(1-b))
  Gain4 : Gain  Gain=1+mNa*(b/(1-b))
  Integrator : Integrator  InitialCondition=Vr
  Sum : Sum  Inputs=|---+
  Sum1 : Sum  Inputs=|++
  HHout : Outport
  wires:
  Sum/1 -> Gain/1
  Gain/1 -> Integrator/1
  FK/1(FKout) -> Gain4/1
  FNa/1(FNaOut) -> Gain2/1
  FL/1 -> Gain3/1
  HHin/1 -> Gain1/1
  Integrator/1 -> Sum1/1
  Sum1/1 -> HHout/1, FNa/1(FNaIn), FL/1, FK/1(FKIn)
  VRefIn/1 -> Sum1/2
  Gain1/1 -> Sum/4
  Gain4/1 -> Sum/1
  Gain2/1 -> Sum/2
  Gain3/1 -> Sum/3

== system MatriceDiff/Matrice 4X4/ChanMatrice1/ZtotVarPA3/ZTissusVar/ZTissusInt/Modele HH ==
  HHin : Inport  Port=1  LatchInput=off
  VRefIn : Inport  Port=2  LatchInput=off
  FK : Subsystem
  FL : Fcn  Expr=gl*(u-Vl)
  FNa : Subsystem
  Gain : Gain  Gain=(1-b)/C
  Gain1 : Gain  Gain=1/(Sm*(1-b))
  Gain2 : Gain  Gain=1+mK*(b/(1-b))
  Gain3 : Gain  Gain=1+mL*(b/(1-b))
  Gain4 : Gain  Gain=1+mNa*(b/(1-b))
  Integrator : Integrator  InitialCondition=Vr
  Sum : Sum  Inputs=|---+
  Sum1 : Sum  Inputs=|+-
  HHout : Outport
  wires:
  Sum/1 -> Gain/1
  Gain/1 -> Integrator/1
  FK/1(FKout) -> Gain4/1
  FNa/1(FNaOut) -> Gain2/1
  FL/1 -> Gain3/1
  HHin/1 -> Gain1/1
  Integrator/1 -> Sum1/1
  Sum1/1 -> HHout/1, FNa/1(FNaIn), FL/1, FK/1(FKIn)
  VRefIn/1 -> Sum1/2
  Gain1/1 -> Sum/4
  Gain4/1 -> Sum/1
  Gain2/1 -> Sum/2
  Gain3/1 -> Sum/3

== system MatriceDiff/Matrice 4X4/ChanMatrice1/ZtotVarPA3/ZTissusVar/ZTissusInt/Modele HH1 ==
  HHin : Inport  Port=1  LatchInput=off
  VRefIn : Inport  Port=2  LatchInput=off
  FK : Subsystem
  FL : Fcn  Expr=gl*(u-Vl)
  FNa : Subsystem
  Gain : Gain  Gain=(1-b)/C
  Gain1 : Gain  Gain=1/(Sm*(1-b))
  Gain2 : Gain  Gain=1+mK*(b/(1-b))
  Gain3 : Gain  Gain=1+mL*(b/(1-b))
  Gain4 : Gain  Gain=1+mNa*(b/(1-b))
  Integrator : Integrator  InitialCondition=Vr
  Sum : Sum  Inputs=|---+
  Sum1 : Sum  Inputs=|++
  HHout : Outport
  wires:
  Sum/1 -> Gain/1
  Gain/1 -> Integrator/1
  FK/1(FKout) -> Gain4/1
  FNa/1(FNaOut) -> Gain2/1
  FL/1 -> Gain3/1
  HHin/1 -> Gain1/1
  Integrator/1 -> Sum1/1
  Sum1/1 -> HHout/1, FNa/1(FNaIn), FL/1, FK/1(FKIn)
  VRefIn/1 -> Sum1/2
  Gain1/1 -> Sum/4
  Gain4/1 -> Sum/1
  Gain2/1 -> Sum/2
  Gain3/1 -> Sum/3

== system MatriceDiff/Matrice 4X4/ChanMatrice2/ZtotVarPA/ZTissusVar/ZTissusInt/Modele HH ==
  HHin : Inport  Port=1  LatchInput=off
  VRefIn : Inport  Port=2  LatchInput=off
  FK : Subsystem
  FL : Fcn  Expr=gl*(u-Vl)
  FNa : Subsystem
  Gain : Gain  Gain=(1-b)/C
  Gain1 : Gain  Gain=1/(Sm*(1-b))
  Gain2 : Gain  Gain=1+mK*(b/(1-b))
  Gain3 : Gain  Gain=1+mL*(b/(1-b))
  Gain4 : Gain  Gain=1+mNa*(b/(1-b))
  Integrator : Integrator  InitialCondition=Vr
  Sum : Sum  Inputs=|---+
  Sum1 : Sum  Inputs=|+-
  HHout : Outport
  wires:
  Sum/1 -> Gain/1
  Gain/1 -> Integrator/1
  FK/1(FKout) -> Gain4/1
  FNa/1(FNaOut) -> Gain2/1
  FL/1 -> Gain3/1
  HHin/1 -> Gain1/1
  Integrator/1 -> Sum1/1
  Sum1/1 -> HHout/1, FNa/1(FNaIn), FL/1, FK/1(FKIn)
  VRefIn/1 -> Sum1/2
  Gain1/1 -> Sum/4
  Gain4/1 -> Sum/1
  Gain2/1 -> Sum/2
  Gain3/1 -> Sum/3

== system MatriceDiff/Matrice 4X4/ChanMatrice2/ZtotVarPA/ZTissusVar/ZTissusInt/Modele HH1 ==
  HHin : Inport  Port=1  LatchInput=off
  VRefIn : Inport  Port=2  LatchInput=off
  FK : Subsystem
  FL : Fcn  Expr=gl*(u-Vl)
  FNa : Subsystem
  Gain : Gain  Gain=(1-b)/C
  Gain1 : Gain  Gain=1/(Sm*(1-b))
  Gain2 : Gain  Gain=1+mK*(b/(1-b))
  Gain3 : Gain  Gain=1+mL*(b/(1-b))
  Gain4 : Gain  Gain=1+mNa*(b/(1-b))
  Integrator : Integrator  InitialCondition=Vr
  Sum : Sum  Inputs=|---+
  Sum1 : Sum  Inputs=|++
  HHout : Outport
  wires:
  Sum/1 -> Gain/1
  Gain/1 -> Integrator/1
  FK/1(FKout) -> Gain4/1
  FNa/1(FNaOut) -> Gain2/1
  FL/1 -> Gain3/1
  HHin/1 -> Gain1/1
  Integrator/1 -> Sum1/1
  Sum1/1 -> HHout/1, FNa/1(FNaIn), FL/1, FK/1(FKIn)
  VRefIn/1 -> Sum1/2
  Gain1/1 -> Sum/4
  Gain4/1 -> Sum/1
  Gain2/1 -> Sum/2
  Gain3/1 -> Sum/3

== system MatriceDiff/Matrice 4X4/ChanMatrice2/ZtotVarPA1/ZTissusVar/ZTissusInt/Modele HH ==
  HHin : Inport  Port=1  LatchInput=off
  VRefIn : Inport  Port=2  LatchInput=off
  FK : Subsystem
  FL : Fcn  Expr=gl*(u-Vl)
  FNa : Subsystem
  Gain : Gain  Gain=(1-b)/C
  Gain1 : Gain  Gain=1/(Sm*(1-b))
  Gain2 : Gain  Gain=1+mK*(b/(1-b))
  Gain3 : Gain  Gain=1+mL*(b/(1-b))
  Gain4 : Gain  Gain=1+mNa*(b/(1-b))
  Integrator : Integrator  InitialCondition=Vr
  Sum : Sum  Inputs=|---+
  Sum1 : Sum  Inputs=|+-
  HHout : Outport
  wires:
  Sum/1 -> Gain/1
  Gain/1 -> Integrator/1
  FK/1(FKout) -> Gain4/1
  FNa/1(FNaOut) -> Gain2/1
  FL/1 -> Gain3/1
  HHin/1 -> Gain1/1
  Integrator/1 -> Sum1/1
  Sum1/1 -> HHout/1, FNa/1(FNaIn), FL/1, FK/1(FKIn)
  VRefIn/1 -> Sum1/2
  Gain1/1 -> Sum/4
  Gain4/1 -> Sum/1
  Gain2/1 -> Sum/2
  Gain3/1 -> Sum/3

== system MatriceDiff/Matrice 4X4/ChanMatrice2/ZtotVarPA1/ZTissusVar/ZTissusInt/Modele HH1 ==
  HHin : Inport  Port=1  LatchInput=off
  VRefIn : Inport  Port=2  LatchInput=off
  FK : Subsystem
  FL : Fcn  Expr=gl*(u-Vl)
  FNa : Subsystem
  Gain : Gain  Gain=(1-b)/C
  Gain1 : Gain  Gain=1/(Sm*(1-b))
  Gain2 : Gain  Gain=1+mK*(b/(1-b))
  Gain3 : Gain  Gain=1+mL*(b/(1-b))
  Gain4 : Gain  Gain=1+mNa*(b/(1-b))
  Integrator : Integrator  InitialCondition=Vr
  Sum : Sum  Inputs=|---+
  Sum1 : Sum  Inputs=|++
  HHout : Outport
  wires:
  Sum/1 -> Gain/1
  Gain/1 -> Integrator/1
  FK/1(FKout) -> Gain4/1
  FNa/1(FNaOut) -> Gain2/1
  FL/1 -> Gain3/1
  HHin/1 -> Gain1/1
  Integrator/1 -> Sum1/1
  Sum1/1 -> HHout/1, FNa/1(FNaIn), FL/1, FK/1(FKIn)
  VRefIn/1 -> Sum1/2
  Gain1/1 -> Sum/4
  Gain4/1 -> Sum/1
  Gain2/1 -> Sum/2
  Gain3/1 -> Sum/3

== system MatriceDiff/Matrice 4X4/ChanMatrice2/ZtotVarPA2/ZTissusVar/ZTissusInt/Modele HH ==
  HHin : Inport  Port=1  LatchInput=off
  VRefIn : Inport  Port=2  LatchInput=off
  FK : Subsystem
  FL : Fcn  Expr=gl*(u-Vl)
  FNa : Subsystem
  Gain : Gain  Gain=(1-b)/C
  Gain1 : Gain  Gain=1/(Sm*(1-b))
  Gain2 : Gain  Gain=1+mK*(b/(1-b))
  Gain3 : Gain  Gain=1+mL*(b/(1-b))
  Gain4 : Gain  Gain=1+mNa*(b/(1-b))
  Integrator : Integrator  InitialCondition=Vr
  Sum : Sum  Inputs=|---+
  Sum1 : Sum  Inputs=|+-
  HHout : Outport
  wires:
  Sum/1 -> Gain/1
  Gain/1 -> Integrator/1
  FK/1(FKout) -> Gain4/1
  FNa/1(FNaOut) -> Gain2/1
  FL/1 -> Gain3/1
  HHin/1 -> Gain1/1
  Integrator/1 -> Sum1/1
  Sum1/1 -> HHout/1, FNa/1(FNaIn), FL/1, FK/1(FKIn)
  VRefIn/1 -> Sum1/2
  Gain1/1 -> Sum/4
  Gain4/1 -> Sum/1
  Gain2/1 -> Sum/2
  Gain3/1 -> Sum/3

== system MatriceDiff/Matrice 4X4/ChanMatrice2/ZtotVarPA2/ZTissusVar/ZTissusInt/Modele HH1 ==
  HHin : Inport  Port=1  LatchInput=off
  VRefIn : Inport  Port=2  LatchInput=off
  FK : Subsystem
  FL : Fcn  Expr=gl*(u-Vl)
  FNa : Subsystem
  Gain : Gain  Gain=(1-b)/C
  Gain1 : Gain  Gain=1/(Sm*(1-b))
  Gain2 : Gain  Gain=1+mK*(b/(1-b))
  Gain3 : Gain  Gain=1+mL*(b/(1-b))
  Gain4 : Gain  Gain=1+mNa*(b/(1-b))
  Integrator : Integrator  InitialCondition=Vr
  Sum : Sum  Inputs=|---+
  Sum1 : Sum  Inputs=|++
  HHout : Outport
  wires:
  Sum/1 -> Gain/1
  Gain/1 -> Integrator/1
  FK/1(FKout) -> Gain4/1
  FNa/1(FNaOut) -> Gain2/1
  FL/1 -> Gain3/1
  HHin/1 -> Gain1/1
  Integrator/1 -> Sum1/1
  Sum1/1 -> HHout/1, FNa/1(FNaIn), FL/1, FK/1(FKIn)
  VRefIn/1 -> Sum1/2
  Gain1/1 -> Sum/4
  Gain4/1 -> Sum/1
  Gain2/1 -> Sum/2
  Gain3/1 -> Sum/3

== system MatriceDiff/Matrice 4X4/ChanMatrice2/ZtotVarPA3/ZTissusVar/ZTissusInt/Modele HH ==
  HHin : Inport  Port=1  LatchInput=off
  VRefIn : Inport  Port=2  LatchInput=off
  FK : Subsystem
  FL : Fcn  Expr=gl*(u-Vl)
  FNa : Subsystem
  Gain : Gain  Gain=(1-b)/C
  Gain1 : Gain  Gain=1/(Sm*(1-b))
  Gain2 : Gain  Gain=1+mK*(b/(1-b))
  Gain3 : Gain  Gain=1+mL*(b/(1-b))
  Gain4 : Gain  Gain=1+mNa*(b/(1-b))
  Integrator : Integrator  InitialCondition=Vr
  Sum : Sum  Inputs=|---+
  Sum1 : Sum  Inputs=|+-
  HHout : Outport
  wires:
  Sum/1 -> Gain/1
  Gain/1 -> Integrator/1
  FK/1(FKout) -> Gain4/1
  FNa/1(FNaOut) -> Gain2/1
  FL/1 -> Gain3/1
  HHin/1 -> Gain1/1
  Integrator/1 -> Sum1/1
  Sum1/1 -> HHout/1, FNa/1(FNaIn), FL/1, FK/1(FKIn)
  VRefIn/1 -> Sum1/2
  Gain1/1 -> Sum/4
  Gain4/1 -> Sum/1
  Gain2/1 -> Sum/2
  Gain3/1 -> Sum/3

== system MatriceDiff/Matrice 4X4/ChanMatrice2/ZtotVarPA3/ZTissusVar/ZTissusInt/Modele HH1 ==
  HHin : Inport  Port=1  LatchInput=off
  VRefIn : Inport  Port=2  LatchInput=off
  FK : Subsystem
  FL : Fcn  Expr=gl*(u-Vl)
  FNa : Subsystem
  Gain : Gain  Gain=(1-b)/C
  Gain1 : Gain  Gain=1/(Sm*(1-b))
  Gain2 : Gain  Gain=1+mK*(b/(1-b))
  Gain3 : Gain  Gain=1+mL*(b/(1-b))
  Gain4 : Gain  Gain=1+mNa*(b/(1-b))
  Integrator : Integrator  InitialCondition=Vr
  Sum : Sum  Inputs=|---+
  Sum1 : Sum  Inputs=|++
  HHout : Outport
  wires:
  Sum/1 -> Gain/1
  Gain/1 -> Integrator/1
  FK/1(FKout) -> Gain4/1
  FNa/1(FNaOut) -> Gain2/1
  FL/1 -> Gain3/1
  HHin/1 -> Gain1/1
  Integrator/1 -> Sum1/1
  Sum1/1 -> HHout/1, FNa/1(FNaIn), FL/1, FK/1(FKIn)
  VRefIn/1 -> Sum1/2
  Gain1/1 -> Sum/4
  Gain4/1 -> Sum/1
  Gain2/1 -> Sum/2
  Gain3/1 -> Sum/3

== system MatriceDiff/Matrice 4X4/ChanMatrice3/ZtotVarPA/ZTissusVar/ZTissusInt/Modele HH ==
  HHin : Inport  Port=1  LatchInput=off
  VRefIn : Inport  Port=2  LatchInput=off
  FK : Subsystem
  FL : Fcn  Expr=gl*(u-Vl)
  FNa : Subsystem
  Gain : Gain  Gain=(1-b)/C
  Gain1 : Gain  Gain=1/(Sm*(1-b))
  Gain2 : Gain  Gain=1+mK*(b/(1-b))
  Gain3 : Gain  Gain=1+mL*(b/(1-b))
  Gain4 : Gain  Gain=1+mNa*(b/(1-b))
  Integrator : Integrator  InitialCondition=Vr
  Sum : Sum  Inputs=|---+
  Sum1 : Sum  Inputs=|+-
  HHout : Outport
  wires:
  Sum/1 -> Gain/1
  Gain/1 -> Integrator/1
  FK/1(FKout) -> Gain4/1
  FNa/1(FNaOut) -> Gain2/1
  FL/1 -> Gain3/1
  HHin/1 -> Gain1/1
  Integrator/1 -> Sum1/1
  Sum1/1 -> HHout/1, FNa/1(FNaIn), FL/1, FK/1(FKIn)
  VRefIn/1 -> Sum1/2
  Gain1/1 -> Sum/4
  Gain4/1 -> Sum/1
  Gain2/1 -> Sum/2
  Gain3/1 -> Sum/3

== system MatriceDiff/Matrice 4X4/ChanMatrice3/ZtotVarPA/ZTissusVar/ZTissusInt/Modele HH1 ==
  HHin : Inport  Port=1  LatchInput=off
  VRefIn : Inport  Port=2  LatchInput=off
  FK : Subsystem
  FL : Fcn  Expr=gl*(u-Vl)
  FNa : Subsystem
  Gain : Gain  Gain=(1-b)/C
  Gain1 : Gain  Gain=1/(Sm*(1-b))
  Gain2 : Gain  Gain=1+mK*(b/(1-b))
  Gain3 : Gain  Gain=1+mL*(b/(1-b))
  Gain4 : Gain  Gain=1+mNa*(b/(1-b))
  Integrator : Integrator  InitialCondition=Vr
  Sum : Sum  Inputs=|---+
  Sum1 : Sum  Inputs=|++
  HHout : Outport
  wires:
  Sum/1 -> Gain/1
  Gain/1 -> Integrator/1
  FK/1(FKout) -> Gain4/1
  FNa/1(FNaOut) -> Gain2/1
  FL/1 -> Gain3/1
  HHin/1 -> Gain1/1
  Integrator/1 -> Sum1/1
  Sum1/1 -> HHout/1, FNa/1(FNaIn), FL/1, FK/1(FKIn)
  VRefIn/1 -> Sum1/2
  Gain1/1 -> Sum/4
  Gain4/1 -> Sum/1
  Gain2/1 -> Sum/2
  Gain3/1 -> Sum/3

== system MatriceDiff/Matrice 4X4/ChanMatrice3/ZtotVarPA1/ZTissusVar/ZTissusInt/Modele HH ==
  HHin : Inport  Port=1  LatchInput=off
  VRefIn : Inport  Port=2  LatchInput=off
  FK : Subsystem
  FL : Fcn  Expr=gl*(u-Vl)
  FNa : Subsystem
  Gain : Gain  Gain=(1-b)/C
  Gain1 : Gain  Gain=1/(Sm*(1-b))
  Gain2 : Gain  Gain=1+mK*(b/(1-b))
  Gain3 : Gain  Gain=1+mL*(b/(1-b))
  Gain4 : Gain  Gain=1+mNa*(b/(1-b))
  Integrator : Integrator  InitialCondition=Vr
  Sum : Sum  Inputs=|---+
  Sum1 : Sum  Inputs=|+-
  HHout : Outport
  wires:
  Sum/1 -> Gain/1
  Gain/1 -> Integrator/1
  FK/1(FKout) -> Gain4/1
  FNa/1(FNaOut) -> Gain2/1
  FL/1 -> Gain3/1
  HHin/1 -> Gain1/1
  Integrator/1 -> Sum1/1
  Sum1/1 -> HHout/1, FNa/1(FNaIn), FL/1, FK/1(FKIn)
  VRefIn/1 -> Sum1/2
  Gain1/1 -> Sum/4
  Gain4/1 -> Sum/1
  Gain2/1 -> Sum/2
  Gain3/1 -> Sum/3
